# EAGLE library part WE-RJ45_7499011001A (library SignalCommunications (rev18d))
Order Code 7499011001A Design THT xBase-T 10/100 Base-T Ports 1x1 Application Standard Tab Position Down LED (Left-Right) NONE EMI Fingers Yes Details see: http://katalog.we-online.de/en/pbs/WE-LAN_RJ45/7499011001A? Updated by Yingchun Shan 2016-08-29 2016(C) Würth Elektronik
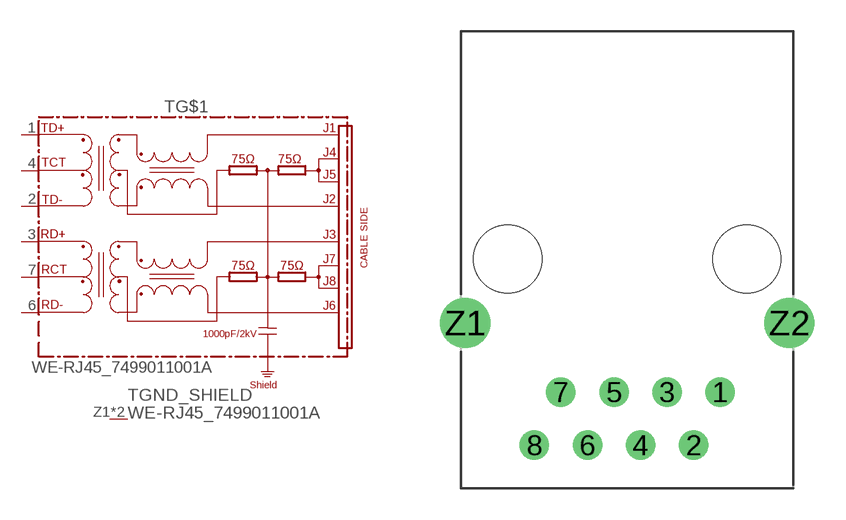
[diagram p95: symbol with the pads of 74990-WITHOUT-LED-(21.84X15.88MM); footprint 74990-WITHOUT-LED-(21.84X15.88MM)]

Designator prefix T; gates GND_SHIELD=GND_PIN G$1=7499011001A

## WE-RJ45_7499011001A (COMPANY-URL: http://www.we-online.de; CREATED-BY: Christin Zierenner; CREATED-DATE: AUG 2012; DATASHEET-URL: http://katalog.we-online.de/kataloge/eisos/media/pdf/7499011001A.pdf; MANUFACTURER: Würth Elektronik eiSos GmbH)  [74990-WITHOUT-LED-(21.84X15.88MM)]
1  G$1:TD+
2  G$1:TD-
3  G$1:RD+
4  G$1:TCT
6  G$1:RD-
7  G$1:RCT
Z1  GND_SHIELD:1  pwr
Z2  GND_SHIELD:1  pwr

## Footprint 74990-WITHOUT-LED-(21.84X15.88MM) (pad centres in mm)
MAX HEIGHT=13.95mm PORTS----1X1 LED ----NO
drill 0.9: 1 4.445,-6.35; 2 3.175,-8.89; 3 1.905,-6.35; 4 0.635,-8.89; 5 -0.635,-6.35; 6 -1.905,-8.89; 7 -3.175,-6.35; 8 -4.445,-8.89
drill 1.6: Z1 -7.745,-3.05; Z2 7.745,-3.05
hole 3.25 at 5.715,0
hole 3.25 at -5.715,0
